(* Logix 5000 AddOnInstructionDefinition export AMCI_5034_PTO_AM_Program_Blend_Move; software revision 37.00 *)

TYPE AMCI_5034_PTO_AM_Input_Data :
STRUCT
   ConnectionFaulted : DINT;
   MovingCW : BOOL;
   MovingCCW : BOOL;
   InHoldState : BOOL;
   Stopped : BOOL;
   AtHome : BOOL;
   Accelerating : BOOL;
   Decelerating : BOOL;
   MoveComplete : BOOL;
   HomeInvalid : BOOL;
   InvalidProfile : BOOL;
   PositionInvalid : BOOL;
   InputError : BOOL;
   CommandError : BOOL;
   ConfigurationError : BOOL;
   ModuleOK : BOOL;
   GeneralPurposeOutputStatus : BOOL;
   Input1Active : BOOL;
   Input2Active : BOOL;
   Input3Active : BOOL;
   Input4Active : BOOL;
   bit_20_reserved : BOOL;
   bit_21_reserved : BOOL;
   bit_22_reserved : BOOL;
   EncoderFollowerMode : BOOL;
   BlendMoveRunning : BOOL;
   BlendMoveAcknowledge : BOOL;
   MinimumRegistrationProgrammed : BOOL;
   EncoderMotionDirection : BOOL;
   MultipleInputsWithSameFunction : BOOL;
   FSCExceedsNumberOfDataBits : BOOL;
   AbsoluteEncoderSetupError : BOOL;
   bit_31_reserved : BOOL;
   CurrentPosition : DINT;
   EncoderPosition : DINT;
   CapturedPosition : DINT;
END_STRUCT
END_TYPE

TYPE AMCI_5034_PTO_AM_Output_Data :
STRUCT
   Command_Word : DINT;
   TargetPosition : DINT;
   TargetVelocity : UDINT;
   Acceleration : DINT;
   Deceleration : DINT;
END_STRUCT
END_TYPE

ADD_ON_INSTRUCTION AMCI_5034_PTO_AM_Program_Blend_Move   (* revision 0.0, ExecuteEnableInFalse *)
// Revision note:
// 10/01/2025 initial release
// Help:
// Programs up to 16 segments of a blend move.
// AXIS INPUT DATA:  Input data from the AMCI 5034-PTO-AM.   Uses the AMCI_5034_PTO_Input_Data User Defined Data Type.
// AXIS OUTPUT DATA; Output data from the AOI to the AMCI 5034-PTO-AM.    Uses the AMCI_5034_PTO_Output_Data User Defined Data Type.
// NUMBER_OF_SEGMENTS: Defines the number of segments in the blend move.   Range of 2 to 16.
// FINAL_MOVE_DECELERATION: Defines the deceleration from the last sement to rest.
// SEGMENT_X_DISTANCE: The relative move distance of each of the segments.
// SEGMENT_X_TARGETVELOCITY: The speed of the segment.
// SEGMENT_X_ ACCELERATION_DECELERATION: The value to accelerate or decelerate from one segment to the next segment.
// EN: Set whe the rung with the Program Blend AOI is receiving power.
// ER: Set when there is a Command Error, Configuation Error, Input Error, or Invalid Profile Error.
// IP: Set when each segment of the blend profile is being programmed.
// BLEND_MOVE_PROGRAMMED: Set when all of the segments of the blend profile have been programmed.
VAR_IN_OUT
   Axis_Input_Data : AMCI_5034_PTO_AM_Input_Data; {required}
   Axis_Output_Data : AMCI_5034_PTO_AM_Output_Data; {required}
END_VAR
VAR_INPUT
   Number_of_Segments : DINT; {required}
   Acceleration_Type_segments_1_to_16 : DINT;
   Final_Move_Deceleration : DINT; {required}
   Segment_1_Distance : DINT; {required}
   Segment_1_TargetVelocity : DINT; {required}
   Segment_1_Acceleration_Deceleration : DINT; {required}
   Segment_2_Distance : DINT; {required}
   Segment_2_TargetVelocity : DINT; {required}
   Segment_2_Acceleration_Deceleration : DINT; {required}
   Segment_3_Distance : DINT; {required}
   Segment_3_TargetVelocity : DINT; {required}
   Segment_3_Acceleration_Deceleration : DINT; {required}
   Segment_4_Distance : DINT; {required}
   Segment_4_TargetVelocity : DINT; {required}
   Segment_4_Acceleration_Deceleration : DINT; {required}
   Segment_5_Distance : DINT; {required}
   Segment_5_TargetVelocity : DINT; {required}
   Segment_5_Acceleration_Deceleration : DINT; {required}
   Segment_6_Distance : DINT; {required}
   Segment_6_TargetVelocity : DINT; {required}
   Segment_6_Acceleration_Deceleration : DINT; {required}
   Segment_7_Distance : DINT; {required}
   Segment_7_TargetVelocity : DINT; {required}
   Segment_7_Acceleration_Deceleration : DINT; {required}
   Segment_8_Distance : DINT; {required}
   Segment_8_TargetVelocity : DINT; {required}
   Segment_8_Acceleration_Deceleration : DINT; {required}
   Segment_9_Distance : DINT; {required}
   Segment_9_TargetVelocity : DINT; {required}
   Segment_9_Acceleration_Deceleration : DINT; {required}
   Segment_10_Distance : DINT; {required}
   Segment_10_TargetVelocity : DINT; {required}
   Segment_10_Acceleration_Deceleration : DINT; {required}
   Segment_11_Distance : DINT; {required}
   Segment_11_TargetVelocity : DINT; {required}
   Segment_11_Acceleration_Deceleration : DINT; {required}
   Segment_12_Distance : DINT; {required}
   Segment_12_TargetVelocity : DINT; {required}
   Segment_12_Acceleration_Deceleration : DINT; {required}
   Segment_13_Distance : DINT; {required}
   Segment_13_TargetVelocity : DINT; {required}
   Segment_13_Acceleration_Deceleration : DINT; {required}
   Segment_14_Distance : DINT; {required}
   Segment_14_TargetVelocity : DINT; {required}
   Segment_14_Acceleration_Deceleration : DINT; {required}
   Segment_15_Distance : DINT; {required}
   Segment_15_TargetVelocity : DINT; {required}
   Segment_15_Acceleration_Deceleration : DINT; {required}
   Segment_16_Distance : DINT; {required}
   Segment_16_TargetVelocity : DINT; {required}
   Segment_16_Acceleration_Deceleration : DINT; {required}
END_VAR
VAR_OUTPUT
   EN : BOOL; {visible}   // set when rung with AOI is true
   ER : BOOL; {visible}   // set when invalid profile, input error, command error, or configuration error
   IP : BOOL; {visible}   // Set when Blend Move is being programmed
   Blend_Move_Programmed : BOOL; {access Read Only, visible}
END_VAR
VAR
   command_data_block : DINT[5];
   Blend_Move_setup : DINT[5];
   Blend_Move_counter : COUNTER;
END_VAR

ROUTINE EnableInFalse   (* ladder *)
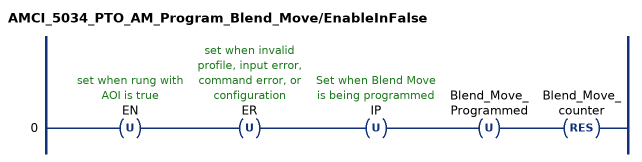
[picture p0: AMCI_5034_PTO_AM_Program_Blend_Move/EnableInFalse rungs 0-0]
   0: OTU(EN)OTU(ER)OTU(IP)OTU(Blend_Move_Programmed)RES(Blend_Move_counter);
END_ROUTINE

ROUTINE Logic   (* ladder *)
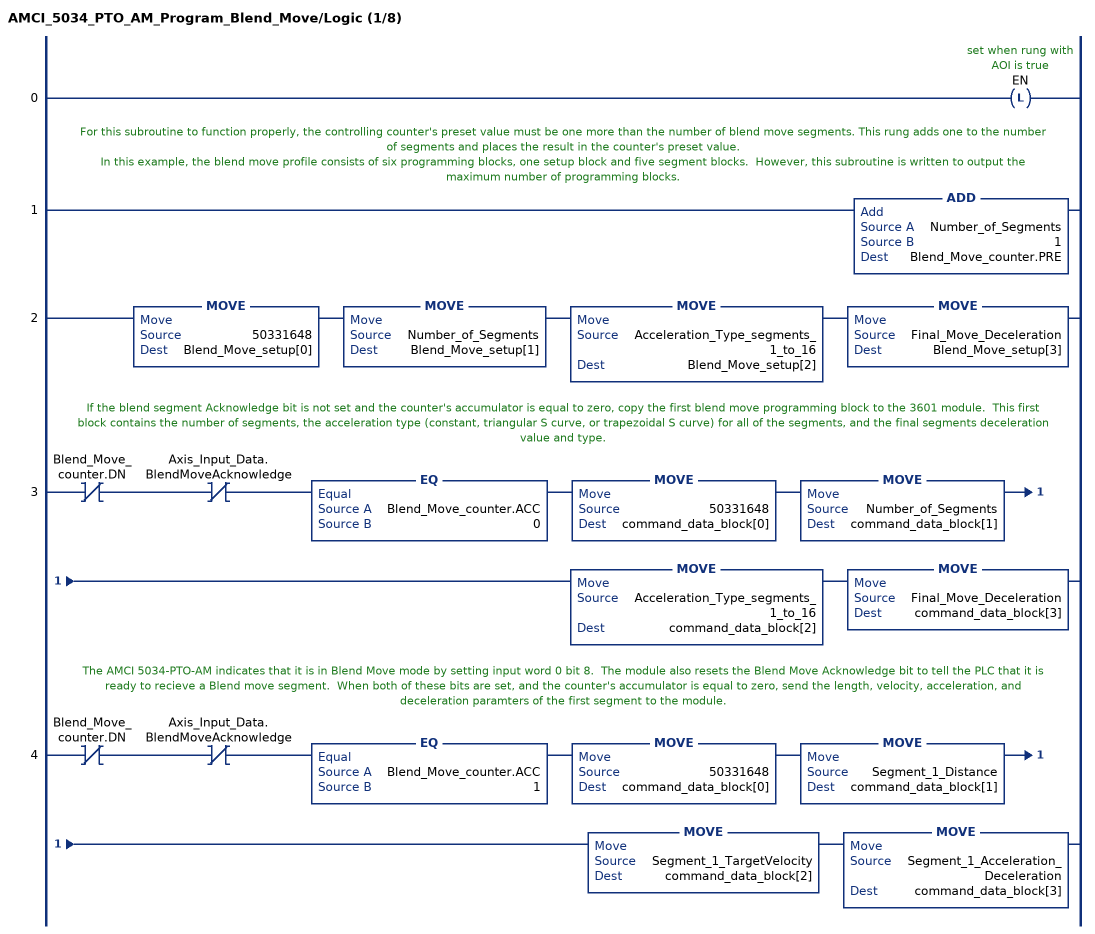
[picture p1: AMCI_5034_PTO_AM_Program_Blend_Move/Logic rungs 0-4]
   0: OTL(EN);
   // For this subroutine to function properly, the controlling counter's preset value must be one more than the number of blend move segments. This rung adds one to the number of segments and places the result in the counter's preset value.
   // In this example, the blend move profile consists of six programming blocks, one setup block and five segment blocks.  However, this subroutine is written to output the maximum number of programming blocks.
   1: ADD(Number_of_Segments,1,Blend_Move_counter.PRE);
   2: MOVE(50331648,Blend_Move_setup[0])MOVE(Number_of_Segments,Blend_Move_setup[1])MOVE(Acceleration_Type_segments_1_to_16,Blend_Move_setup[2])MOVE(Final_Move_Deceleration,Blend_Move_setup[3]);
   // If the blend segment Acknowledge bit is not set and the counter's accumulator is equal to zero, copy the first blend move programming block to the 3601 module.  This first block contains the number of segments, the acceleration type (constant, triangular S curve, or trapezoidal S curve) for all of the segments, and the final segments deceleration value and type.
   3: XIO(Blend_Move_counter.DN)XIO(Axis_Input_Data.BlendMoveAcknowledge)EQ(Blend_Move_counter.ACC,0)MOVE(50331648,command_data_block[0])MOVE(Number_of_Segments,command_data_block[1])MOVE(Acceleration_Type_segments_1_to_16,command_data_block[2])MOVE(Final_Move_Deceleration,command_data_block[3]);
   // The AMCI 5034-PTO-AM indicates that it is in Blend Move mode by setting input word 0 bit 8.  The module also resets the Blend Move Acknowledge bit to tell the PLC that it is ready to recieve a Blend move segment.  When both of these bits are set, and the counter's accumulator is equal to zero, send the length, velocity, acceleration, and deceleration paramters of the first segment to the module.
   4: XIO(Blend_Move_counter.DN)XIO(Axis_Input_Data.BlendMoveAcknowledge)EQ(Blend_Move_counter.ACC,1)MOVE(50331648,command_data_block[0])MOVE(Segment_1_Distance,command_data_block[1])MOVE(Segment_1_TargetVelocity,command_data_block[2])MOVE(Segment_1_Acceleration_Deceleration,command_data_block[3]);
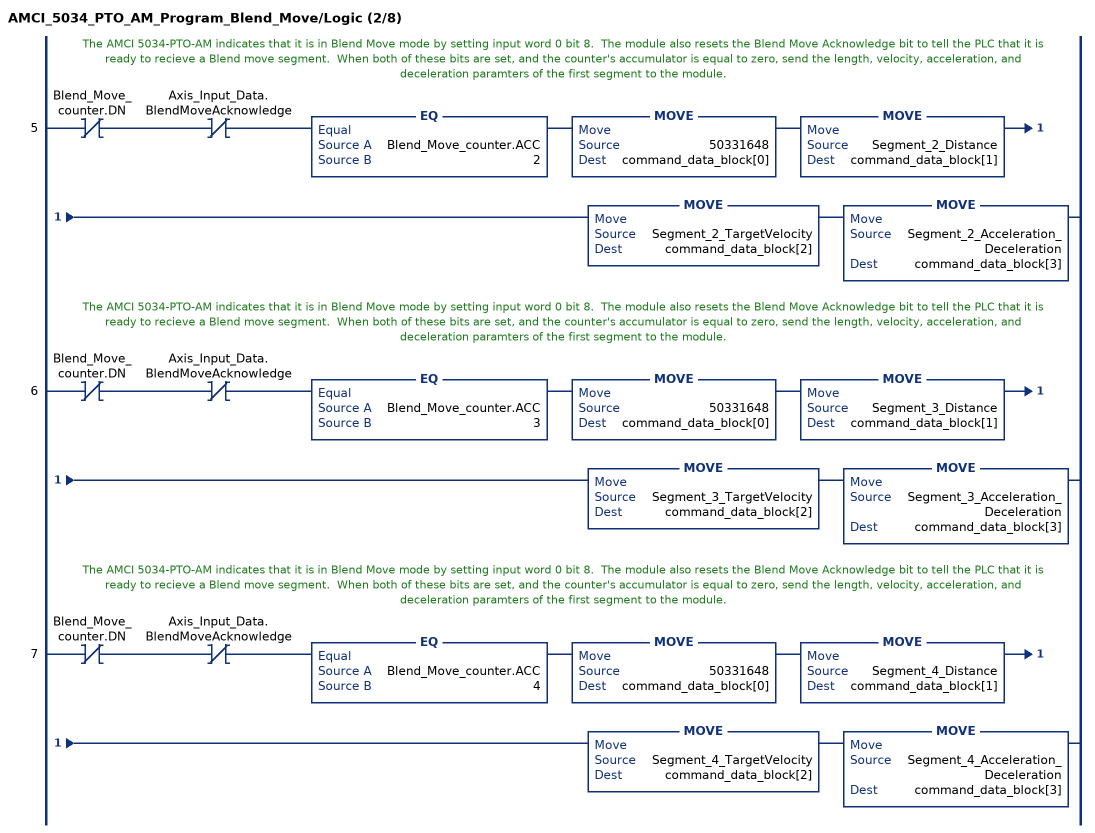
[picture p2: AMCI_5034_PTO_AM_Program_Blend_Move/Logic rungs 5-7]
   // The AMCI 5034-PTO-AM indicates that it is in Blend Move mode by setting input word 0 bit 8.  The module also resets the Blend Move Acknowledge bit to tell the PLC that it is ready to recieve a Blend move segment.  When both of these bits are set, and the counter's accumulator is equal to zero, send the length, velocity, acceleration, and deceleration paramters of the first segment to the module.
   5: XIO(Blend_Move_counter.DN)XIO(Axis_Input_Data.BlendMoveAcknowledge)EQ(Blend_Move_counter.ACC,2)MOVE(50331648,command_data_block[0])MOVE(Segment_2_Distance,command_data_block[1])MOVE(Segment_2_TargetVelocity,command_data_block[2])MOVE(Segment_2_Acceleration_Deceleration,command_data_block[3]);
   // The AMCI 5034-PTO-AM indicates that it is in Blend Move mode by setting input word 0 bit 8.  The module also resets the Blend Move Acknowledge bit to tell the PLC that it is ready to recieve a Blend move segment.  When both of these bits are set, and the counter's accumulator is equal to zero, send the length, velocity, acceleration, and deceleration paramters of the first segment to the module.
   6: XIO(Blend_Move_counter.DN)XIO(Axis_Input_Data.BlendMoveAcknowledge)EQ(Blend_Move_counter.ACC,3)MOVE(50331648,command_data_block[0])MOVE(Segment_3_Distance,command_data_block[1])MOVE(Segment_3_TargetVelocity,command_data_block[2])MOVE(Segment_3_Acceleration_Deceleration,command_data_block[3]);
   // The AMCI 5034-PTO-AM indicates that it is in Blend Move mode by setting input word 0 bit 8.  The module also resets the Blend Move Acknowledge bit to tell the PLC that it is ready to recieve a Blend move segment.  When both of these bits are set, and the counter's accumulator is equal to zero, send the length, velocity, acceleration, and deceleration paramters of the first segment to the module.
   7: XIO(Blend_Move_counter.DN)XIO(Axis_Input_Data.BlendMoveAcknowledge)EQ(Blend_Move_counter.ACC,4)MOVE(50331648,command_data_block[0])MOVE(Segment_4_Distance,command_data_block[1])MOVE(Segment_4_TargetVelocity,command_data_block[2])MOVE(Segment_4_Acceleration_Deceleration,command_data_block[3]);
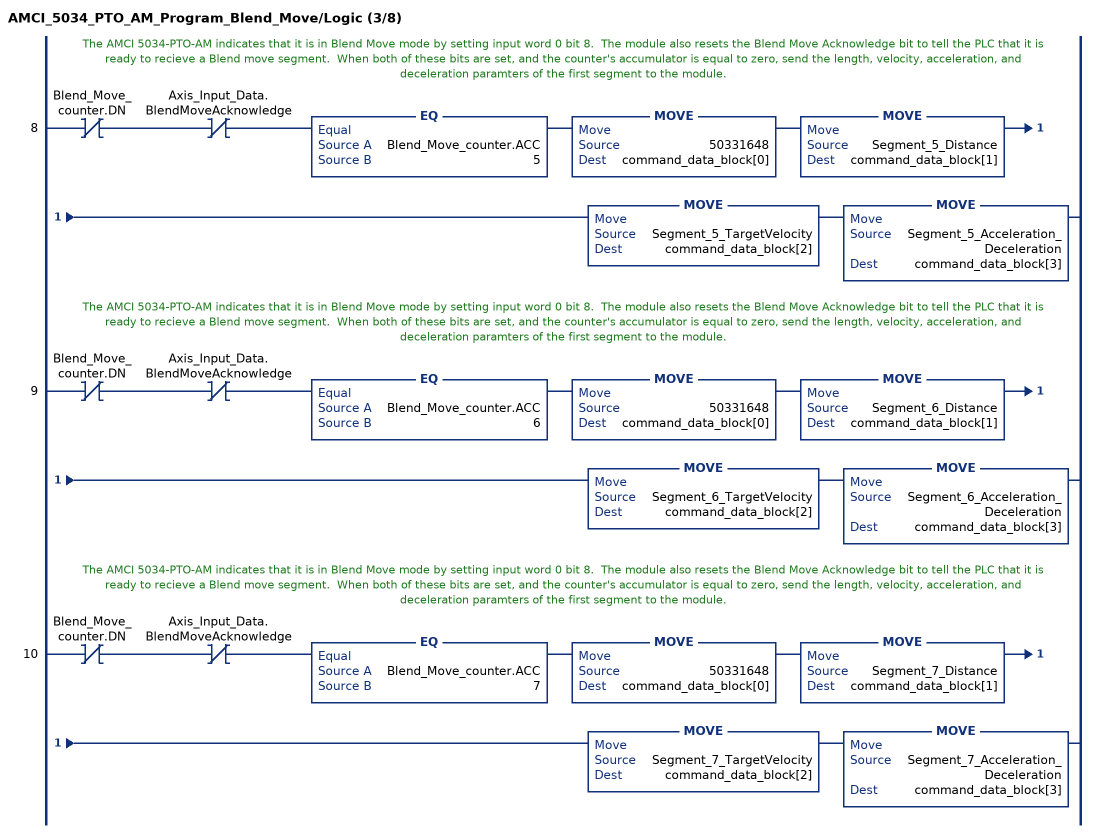
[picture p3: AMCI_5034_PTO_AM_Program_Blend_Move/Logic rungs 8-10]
   // The AMCI 5034-PTO-AM indicates that it is in Blend Move mode by setting input word 0 bit 8.  The module also resets the Blend Move Acknowledge bit to tell the PLC that it is ready to recieve a Blend move segment.  When both of these bits are set, and the counter's accumulator is equal to zero, send the length, velocity, acceleration, and deceleration paramters of the first segment to the module.
   8: XIO(Blend_Move_counter.DN)XIO(Axis_Input_Data.BlendMoveAcknowledge)EQ(Blend_Move_counter.ACC,5)MOVE(50331648,command_data_block[0])MOVE(Segment_5_Distance,command_data_block[1])MOVE(Segment_5_TargetVelocity,command_data_block[2])MOVE(Segment_5_Acceleration_Deceleration,command_data_block[3]);
   // The AMCI 5034-PTO-AM indicates that it is in Blend Move mode by setting input word 0 bit 8.  The module also resets the Blend Move Acknowledge bit to tell the PLC that it is ready to recieve a Blend move segment.  When both of these bits are set, and the counter's accumulator is equal to zero, send the length, velocity, acceleration, and deceleration paramters of the first segment to the module.
   9: XIO(Blend_Move_counter.DN)XIO(Axis_Input_Data.BlendMoveAcknowledge)EQ(Blend_Move_counter.ACC,6)MOVE(50331648,command_data_block[0])MOVE(Segment_6_Distance,command_data_block[1])MOVE(Segment_6_TargetVelocity,command_data_block[2])MOVE(Segment_6_Acceleration_Deceleration,command_data_block[3]);
   // The AMCI 5034-PTO-AM indicates that it is in Blend Move mode by setting input word 0 bit 8.  The module also resets the Blend Move Acknowledge bit to tell the PLC that it is ready to recieve a Blend move segment.  When both of these bits are set, and the counter's accumulator is equal to zero, send the length, velocity, acceleration, and deceleration paramters of the first segment to the module.
   10: XIO(Blend_Move_counter.DN)XIO(Axis_Input_Data.BlendMoveAcknowledge)EQ(Blend_Move_counter.ACC,7)MOVE(50331648,command_data_block[0])MOVE(Segment_7_Distance,command_data_block[1])MOVE(Segment_7_TargetVelocity,command_data_block[2])MOVE(Segment_7_Acceleration_Deceleration,command_data_block[3]);
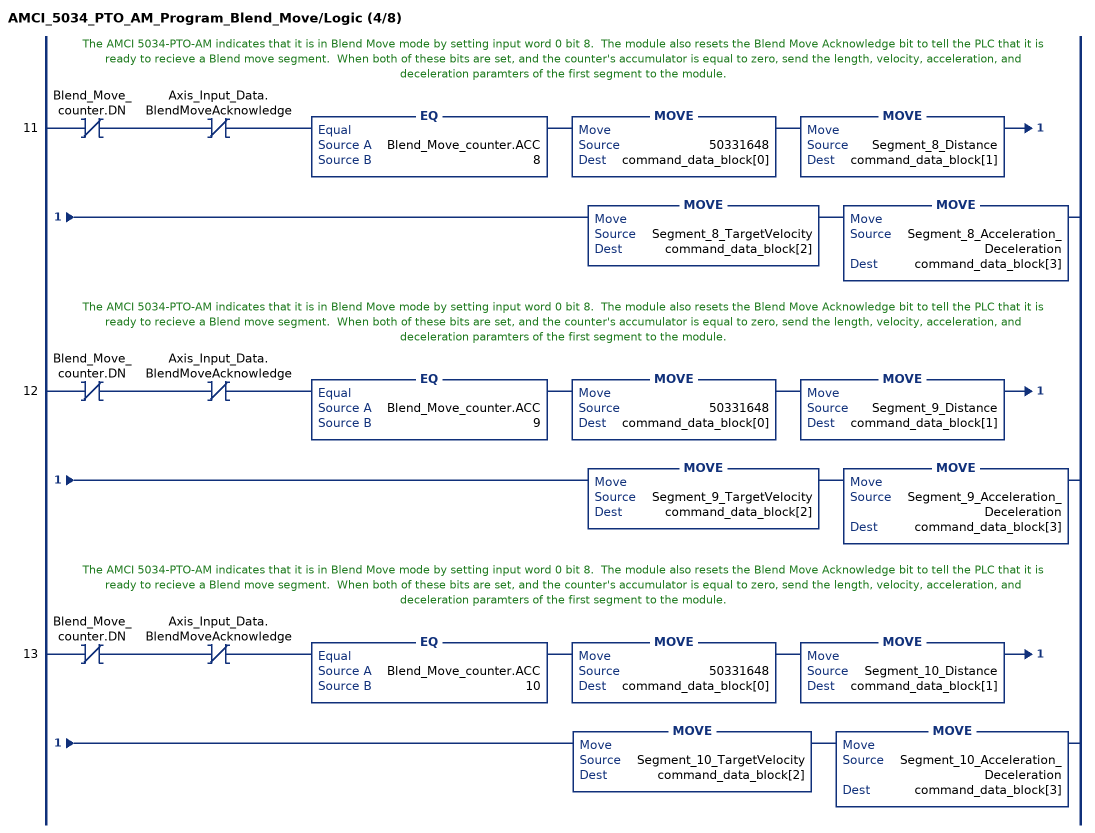
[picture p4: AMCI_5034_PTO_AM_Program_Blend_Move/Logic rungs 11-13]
   // The AMCI 5034-PTO-AM indicates that it is in Blend Move mode by setting input word 0 bit 8.  The module also resets the Blend Move Acknowledge bit to tell the PLC that it is ready to recieve a Blend move segment.  When both of these bits are set, and the counter's accumulator is equal to zero, send the length, velocity, acceleration, and deceleration paramters of the first segment to the module.
   11: XIO(Blend_Move_counter.DN)XIO(Axis_Input_Data.BlendMoveAcknowledge)EQ(Blend_Move_counter.ACC,8)MOVE(50331648,command_data_block[0])MOVE(Segment_8_Distance,command_data_block[1])MOVE(Segment_8_TargetVelocity,command_data_block[2])MOVE(Segment_8_Acceleration_Deceleration,command_data_block[3]);
   // The AMCI 5034-PTO-AM indicates that it is in Blend Move mode by setting input word 0 bit 8.  The module also resets the Blend Move Acknowledge bit to tell the PLC that it is ready to recieve a Blend move segment.  When both of these bits are set, and the counter's accumulator is equal to zero, send the length, velocity, acceleration, and deceleration paramters of the first segment to the module.
   12: XIO(Blend_Move_counter.DN)XIO(Axis_Input_Data.BlendMoveAcknowledge)EQ(Blend_Move_counter.ACC,9)MOVE(50331648,command_data_block[0])MOVE(Segment_9_Distance,command_data_block[1])MOVE(Segment_9_TargetVelocity,command_data_block[2])MOVE(Segment_9_Acceleration_Deceleration,command_data_block[3]);
   // The AMCI 5034-PTO-AM indicates that it is in Blend Move mode by setting input word 0 bit 8.  The module also resets the Blend Move Acknowledge bit to tell the PLC that it is ready to recieve a Blend move segment.  When both of these bits are set, and the counter's accumulator is equal to zero, send the length, velocity, acceleration, and deceleration paramters of the first segment to the module.
   13: XIO(Blend_Move_counter.DN)XIO(Axis_Input_Data.BlendMoveAcknowledge)EQ(Blend_Move_counter.ACC,10)MOVE(50331648,command_data_block[0])MOVE(Segment_10_Distance,command_data_block[1])MOVE(Segment_10_TargetVelocity,command_data_block[2])MOVE(Segment_10_Acceleration_Deceleration,command_data_block[3]);
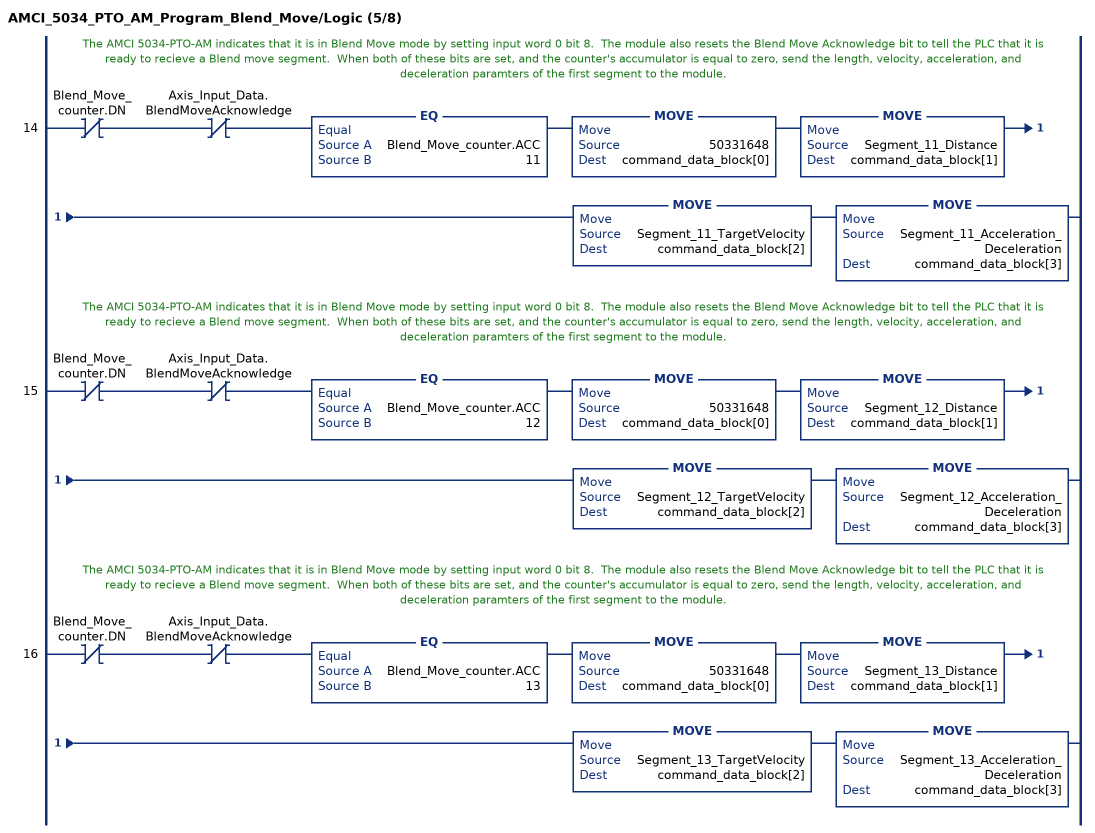
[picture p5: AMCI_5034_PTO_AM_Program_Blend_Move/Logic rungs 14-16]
   // The AMCI 5034-PTO-AM indicates that it is in Blend Move mode by setting input word 0 bit 8.  The module also resets the Blend Move Acknowledge bit to tell the PLC that it is ready to recieve a Blend move segment.  When both of these bits are set, and the counter's accumulator is equal to zero, send the length, velocity, acceleration, and deceleration paramters of the first segment to the module.
   14: XIO(Blend_Move_counter.DN)XIO(Axis_Input_Data.BlendMoveAcknowledge)EQ(Blend_Move_counter.ACC,11)MOVE(50331648,command_data_block[0])MOVE(Segment_11_Distance,command_data_block[1])MOVE(Segment_11_TargetVelocity,command_data_block[2])MOVE(Segment_11_Acceleration_Deceleration,command_data_block[3]);
   // The AMCI 5034-PTO-AM indicates that it is in Blend Move mode by setting input word 0 bit 8.  The module also resets the Blend Move Acknowledge bit to tell the PLC that it is ready to recieve a Blend move segment.  When both of these bits are set, and the counter's accumulator is equal to zero, send the length, velocity, acceleration, and deceleration paramters of the first segment to the module.
   15: XIO(Blend_Move_counter.DN)XIO(Axis_Input_Data.BlendMoveAcknowledge)EQ(Blend_Move_counter.ACC,12)MOVE(50331648,command_data_block[0])MOVE(Segment_12_Distance,command_data_block[1])MOVE(Segment_12_TargetVelocity,command_data_block[2])MOVE(Segment_12_Acceleration_Deceleration,command_data_block[3]);
   // The AMCI 5034-PTO-AM indicates that it is in Blend Move mode by setting input word 0 bit 8.  The module also resets the Blend Move Acknowledge bit to tell the PLC that it is ready to recieve a Blend move segment.  When both of these bits are set, and the counter's accumulator is equal to zero, send the length, velocity, acceleration, and deceleration paramters of the first segment to the module.
   16: XIO(Blend_Move_counter.DN)XIO(Axis_Input_Data.BlendMoveAcknowledge)EQ(Blend_Move_counter.ACC,13)MOVE(50331648,command_data_block[0])MOVE(Segment_13_Distance,command_data_block[1])MOVE(Segment_13_TargetVelocity,command_data_block[2])MOVE(Segment_13_Acceleration_Deceleration,command_data_block[3]);
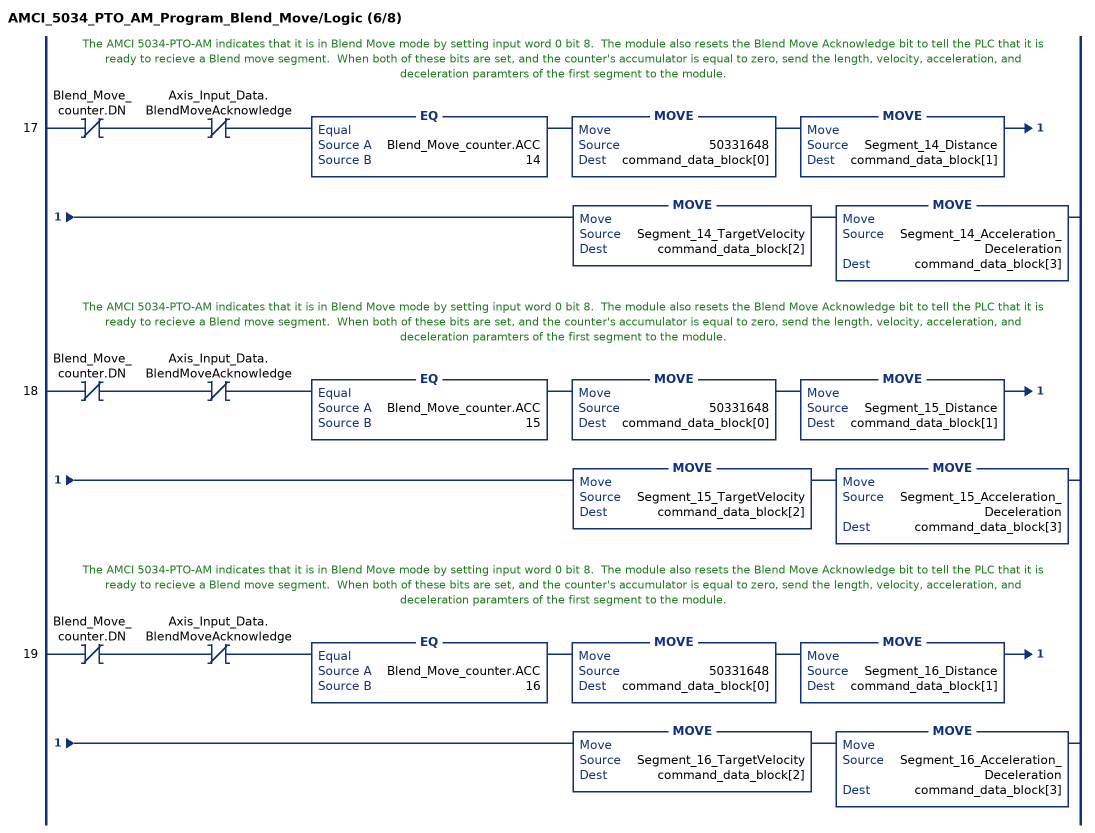
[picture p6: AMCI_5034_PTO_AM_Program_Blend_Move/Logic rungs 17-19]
   // The AMCI 5034-PTO-AM indicates that it is in Blend Move mode by setting input word 0 bit 8.  The module also resets the Blend Move Acknowledge bit to tell the PLC that it is ready to recieve a Blend move segment.  When both of these bits are set, and the counter's accumulator is equal to zero, send the length, velocity, acceleration, and deceleration paramters of the first segment to the module.
   17: XIO(Blend_Move_counter.DN)XIO(Axis_Input_Data.BlendMoveAcknowledge)EQ(Blend_Move_counter.ACC,14)MOVE(50331648,command_data_block[0])MOVE(Segment_14_Distance,command_data_block[1])MOVE(Segment_14_TargetVelocity,command_data_block[2])MOVE(Segment_14_Acceleration_Deceleration,command_data_block[3]);
   // The AMCI 5034-PTO-AM indicates that it is in Blend Move mode by setting input word 0 bit 8.  The module also resets the Blend Move Acknowledge bit to tell the PLC that it is ready to recieve a Blend move segment.  When both of these bits are set, and the counter's accumulator is equal to zero, send the length, velocity, acceleration, and deceleration paramters of the first segment to the module.
   18: XIO(Blend_Move_counter.DN)XIO(Axis_Input_Data.BlendMoveAcknowledge)EQ(Blend_Move_counter.ACC,15)MOVE(50331648,command_data_block[0])MOVE(Segment_15_Distance,command_data_block[1])MOVE(Segment_15_TargetVelocity,command_data_block[2])MOVE(Segment_15_Acceleration_Deceleration,command_data_block[3]);
   // The AMCI 5034-PTO-AM indicates that it is in Blend Move mode by setting input word 0 bit 8.  The module also resets the Blend Move Acknowledge bit to tell the PLC that it is ready to recieve a Blend move segment.  When both of these bits are set, and the counter's accumulator is equal to zero, send the length, velocity, acceleration, and deceleration paramters of the first segment to the module.
   19: XIO(Blend_Move_counter.DN)XIO(Axis_Input_Data.BlendMoveAcknowledge)EQ(Blend_Move_counter.ACC,16)MOVE(50331648,command_data_block[0])MOVE(Segment_16_Distance,command_data_block[1])MOVE(Segment_16_TargetVelocity,command_data_block[2])MOVE(Segment_16_Acceleration_Deceleration,command_data_block[3]);
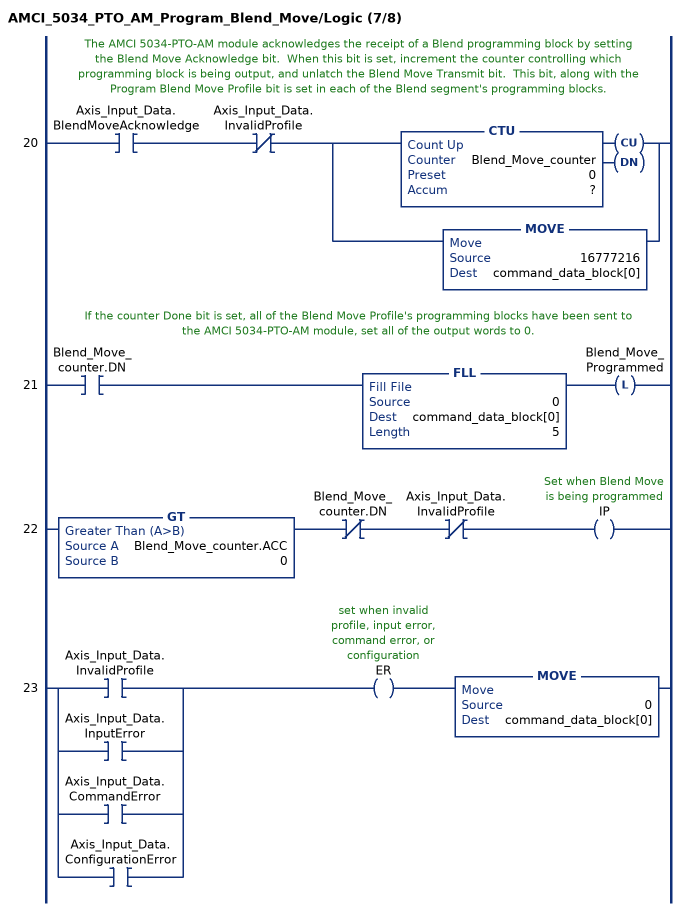
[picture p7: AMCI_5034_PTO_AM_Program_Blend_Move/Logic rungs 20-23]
   // The AMCI 5034-PTO-AM module acknowledges the receipt of a Blend programming block by setting the Blend Move Acknowledge bit.  When this bit is set, increment the counter controlling which programming block is being output, and unlatch the Blend Move Transmit bit.  This bit, along with the Program Blend Move Profile bit is set in each of the Blend segment's programming blocks.
   20: XIC(Axis_Input_Data.BlendMoveAcknowledge)XIO(Axis_Input_Data.InvalidProfile)[CTU(Blend_Move_counter,?,?) ,MOVE(16777216,command_data_block[0]) ];
   // If the counter Done bit is set, all of the Blend Move Profile's programming blocks have been sent to the AMCI 5034-PTO-AM module, set all of the output words to 0.
   21: XIC(Blend_Move_counter.DN)FLL(0,command_data_block[0],5)OTL(Blend_Move_Programmed);
   22: GT(Blend_Move_counter.ACC,0)XIO(Blend_Move_counter.DN)XIO(Axis_Input_Data.InvalidProfile)OTE(IP);
   23: [XIC(Axis_Input_Data.InvalidProfile) ,XIC(Axis_Input_Data.InputError) ,XIC(Axis_Input_Data.CommandError) ,XIC(Axis_Input_Data.ConfigurationError) ]OTE(ER)MOVE(0,command_data_block[0]);
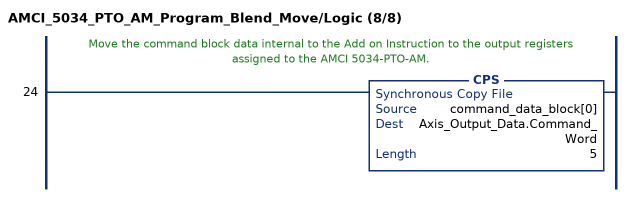
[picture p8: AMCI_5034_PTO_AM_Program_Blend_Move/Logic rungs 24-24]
   // Move the command block data internal to the Add on Instruction to the output registers assigned to the AMCI 5034-PTO-AM.
   24: CPS(command_data_block[0],Axis_Output_Data.Command_Word,5);
END_ROUTINE
END_ADD_ON_INSTRUCTION
